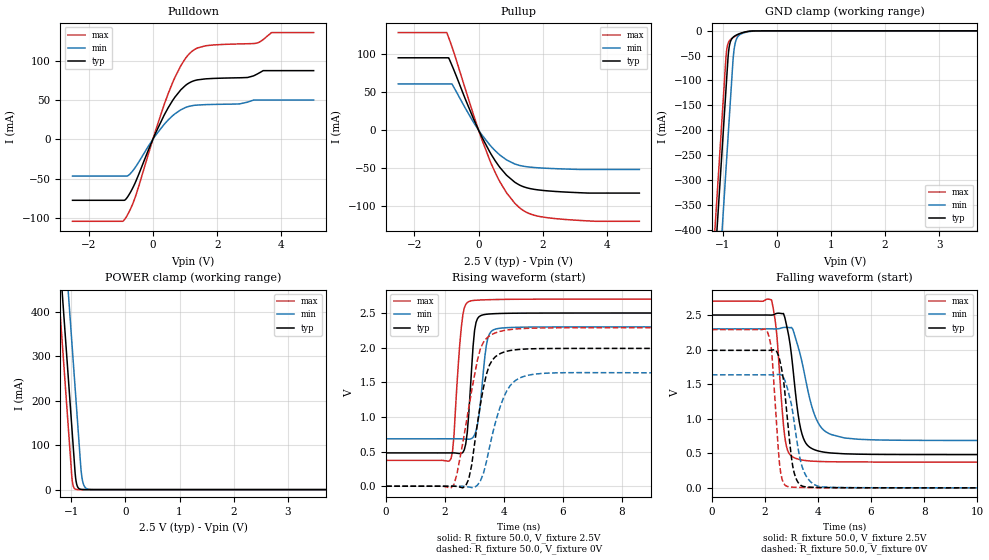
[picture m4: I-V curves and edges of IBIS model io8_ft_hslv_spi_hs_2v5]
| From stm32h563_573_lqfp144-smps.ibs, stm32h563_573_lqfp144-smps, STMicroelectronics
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[Model]   io8_ft_hslv_spi_hs_2v5
Model_type I/O
Polarity   Non-Inverting
Enable   Active-Low
| CAP_THRESHOLD on pad IOFT is "UDTCAPC" :
| Rising=20.0% of vddiom   Falling=80.0% of vddiom
| C_comp min and max val. don't necessarily correlate with the min and max pvt
| but are the smallest and greatest pad capacitance found.
| var   typ   min   max
C_comp   4.85183pF  4.77587pF  4.93407pF
|C_comp_pullup   3.10510pF  2.91245pF  2.94040pF
|C_comp_pulldown   1.74673pF  1.86342pF  1.99367pF
Vinl = 690.0mV
Vinh = 1.89V
Vmeas = 1.25V   | Reference voltage for timing measurements
Cref  = 50.0pF   | Timing specification test load capacitance value
Rref  = 100.0MOhm   | Timing specification test load resistance value
Vref  = 1.25V   | Timing specification test load voltage
[Model Spec]
| TIME_THRESHOLD on pin ZIV11 is "CMOS" :
| Rising=40.0% of vdd   Falling=60.0% of vdd
Vinl 989.80000mV 917.80000mV 1.06580V
Vinh 1.40320V 1.29620V 1.49120V
| variable   typ   min   max
[Temperature Range] 25.0 125.0 -40.0
| variable   typ   min   max
[Voltage Range] 2.5V 2.3V 2.7V
| variable   typ   min   max
[POWER Clamp Reference] 2.5V 2.3V 2.7V
| variable   typ   min   max
[GND Clamp Reference] 0V 0V 0V
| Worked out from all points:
|   slope of the pulldown table from 0 to 0.375 V, typ, clamps not added: 11.5 ohm
|   slope of the pullup table from 0 to 0.375 V, typ, clamps not added: 12.3 ohm
|   GND clamp passes 1 mA (typ) near -0.52 V on its own axis
|   POWER clamp passes 1 mA (typ) near -0.84 V on its own axis
|   rising waveform, R_fixture 50.0, V_fixture 2.5V: 20-80 % time 194ps typ, 239ps min, 222ps max; typ from 0.481 V to 2.5 V
|   falling waveform, R_fixture 50.0, V_fixture 2.5V: 20-80 % time 390ps typ, 626ps min, 277ps max; typ from 2.5 V to 0.481 V
|   rising waveform, R_fixture 50.0, V_fixture 0V: 20-80 % time 458ps typ, 629ps min, 576ps max; typ from 0 V to 1.99 V
|   falling waveform, R_fixture 50.0, V_fixture 0V: 20-80 % time 328ps typ, 451ps min, 244ps max; typ from 1.99 V to 0 V
[POWER Clamp]
-2.5V     2.708A     2.899A     2.597A
-1.23V    548.8mA    740.2mA    437.5mA
-1.16V    429.8mA    621.2mA    318.5mA
-1.07V    276.8mA    468.2mA    165.5mA
-1.03V    208.8mA    400.2mA    97.53mA
-980mV    123.8mA    315.2mA    17.95mA
-920mV    26.3mA     213.2mA    906uA
-880mV    5.543mA    145.2mA    123.7uA
-810mV    363.5uA    33.6mA     3.797uA
-770mV    76.62uA    10.47mA    518.9nA
-700mV    5.026uA    1.361mA    16.14nA
5V        0A         0A         0A
[GND Clamp]
-2.5V     -2.771A    -2.933A    -2.706A
-1.21V    -578.3mA   -739.7mA   -512.8mA
-950mV    -136.3mA   -297.7mA   -70.75mA
-930mV    -102.3mA   -263.7mA   -41.56mA
-900mV    -51.97mA   -212.7mA   -25.14mA
-880mV    -32.59mA   -178.7mA   -20.84mA
-850mV    -19.78mA   -127.7mA   -17.15mA
-810mV    -13.22mA   -60.17mA   -13.75mA
-780mV    -10.64mA   -30.96mA   -11.62mA
-730mV    -7.637mA   -13.21mA   -8.533mA
-430mV    -217.7uA   -562.2uA   -113.2uA
5V        7.27nA     1.305uA    342.4pA
| variable   typ   min   max
[Pullup Reference] 2.5V 2.3V 2.7V
| variable   typ   min   max
[Pulldown Reference] 0V 0V 0V
[Pullup]
-2.5V     94.96mA    60.75mA    128.1mA
-990mV    94.96mA    60.75mA    128.1mA
-930mV    94.96mA    60.75mA    121.3mA
-830mV    85.15mA    60.75mA    109.6mA
-170mV    16.03mA    11.13mA    21.65mA
350mV     -28.74mA   -19.44mA   -39.66mA
610mV     -45.85mA   -30.67mA   -63.5mA
870mV     -59.1mA    -39.02mA   -82.25mA
1.29V     -72.3mA    -46.39mA   -102.3mA
1.64V     -76.94mA   -48.61mA   -110.4mA
2.27V     -80.02mA   -50.27mA   -115.5mA
5V        -82.5mA    -51.48mA   -119.5mA
[Pulldown]
-2.5V     -77.63mA   -46.84mA   -104.3mA
-870mV    -77.25mA   -46.84mA   -101.4mA
-550mV    -55.3mA    -35.88mA   -73.72mA
90mV      8.401mA    5.299mA    11.79mA
610mV     49.03mA    29.76mA    71.69mA
870mV     62.92mA    37.48mA    93.62mA
1.23V     73.63mA    42.72mA    112.2mA
1.64V     76.78mA    44.01mA    118.8mA
2.94V     78.48mA    47.15mA    121.4mA
3.24V     82.82mA    49.81mA    122.4mA
3.69V     87.21mA    49.81mA    135.6mA
5V        87.21mA    49.81mA    135.6mA
[Ramp]
dV/dt_r 1.19346V/454.84718ps 980.82492mV/625.24029ps 1.37306V/574.68247ps
dV/dt_f 1.21165V/388.01181ps 969.25758mV/624.82306ps 1.39628V/274.05095ps
R_load = 50.0
| Removed startup time: 0s 0s 0s  .
| Removed end time: 14.4ns.
[Rising Waveform]
R_fixture   = 50.0
V_fixture   = 2.5V
V_fixture_min = 2.3V
V_fixture_max = 2.7V
0s        480.6mV    684.6mV    372.9mV
2.2ns     480.8mV    684.7mV    399mV
2.3ns     480.9mV    684.9mV    722.7mV
2.55ns    473.7mV    684.6mV    2.292V
2.7ns     609.4mV    679.6mV    2.624V
2.8ns     1.032V     678.3mV    2.664V
3.05ns    2.365V     799.5mV    2.684V
3.4ns     2.482V     2.036V     2.691V
3.7ns     2.49V      2.266V     2.694V
14.4ns    2.5V       2.3V       2.7V
| Removed startup time: 0s 0s 0s  .
| Removed end time: 24.4ns.
[Falling Waveform]
R_fixture   = 50.0
V_fixture   = 2.5V
V_fixture_min = 2.3V
V_fixture_max = 2.7V
0s        2.5V       2.3V       2.7V
2.25ns    2.499V     2.3V       2.718V
2.45ns    2.524V     2.3V       2.207V
2.65ns    2.519V     2.316V     1.131V
2.8ns     2.378V     2.321V     617.7mV
3.3ns     944.2mV    1.973V     410.3mV
3.55ns    642.2mV    1.536V     394.3mV
4ns       534.8mV    945.6mV    382.3mV
5ns       492.5mV    721.5mV    375.5mV
24.4ns    480.6mV    684.6mV    372.9mV
| Removed startup time: 0s 0s 0s  .
| Removed end time: 24.3ns.
[Rising Waveform]
R_fixture   = 50.0
V_fixture   = 0V
V_fixture_min = 0V
V_fixture_max = 0V
0s        101.5nV    479.1nV    83.44nV
2.2ns     112.9uV    -70.04uV   -22.12mV
2.7ns     7.755mV    -3.631mV   873.4mV
2.9ns     301.5mV    -19.17mV   1.374V
3.2ns     1.187V     78.94mV    1.988V
3.5ns     1.744V     549.4mV    2.167V
3.9ns     1.92V      1.186V     2.238V
4.4ns     1.97V      1.53V      2.269V
5.4ns     1.987V     1.63V      2.285V
24.3ns    1.989V     1.635V     2.288V
| Removed startup time: 0s 0s 0s  .
| Removed end time: 24.4ns.
[Falling Waveform]
R_fixture   = 50.0
V_fixture   = 0V
V_fixture_min = 0V
V_fixture_max = 0V
0s        1.989V     1.635V     2.288V
2.1ns     1.989V     1.635V     2.252V
2.25ns    1.992V     1.635V     2V
2.55ns    1.861V     1.64V      348.1mV
2.85ns    987.9mV    1.435V     20.45mV
3.05ns    311mV      1.089V     9.9mV
3.2ns     111.9mV    694.3mV    7.344mV
3.5ns     16.67mV    210.4mV    4.93mV
4.1ns     5.289mV    16.28mV    2.759mV
24.4ns    1.113uV    6.433uV    156.6nV
